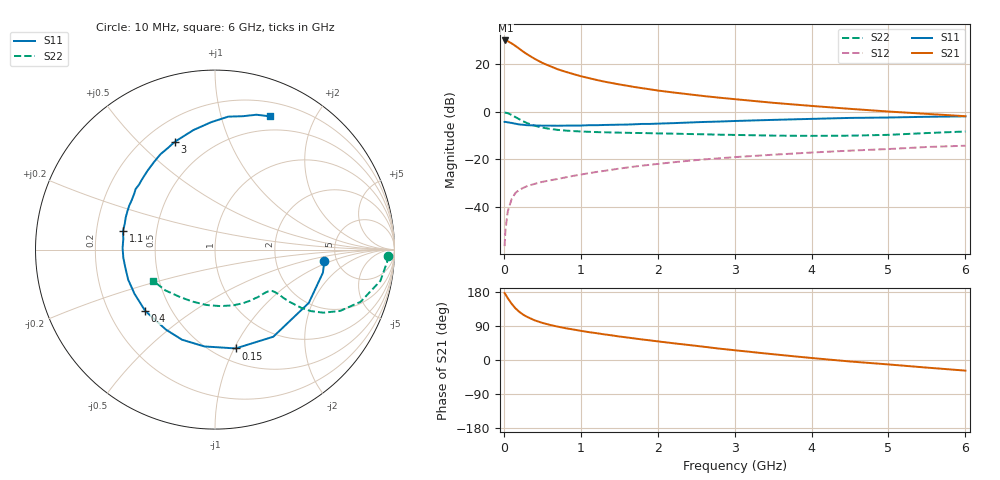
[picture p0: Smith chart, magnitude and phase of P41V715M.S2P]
! SIEMENS Small Signal Semiconductors
! BFP182
! Si NPN RF Bipolar Junction Transistor in SOT143
! VCE = 1.75 V  IC = 15 mA
! Common Emitter S-Parameters:  March  1996
# GHz  S  MA  R  50
!  f  S11  S21  S12  S22
! GHz  MAG  ANG  MAG  ANG  MAG  ANG  MAG  ANG
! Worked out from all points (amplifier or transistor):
!   36 points, 10 MHz to 6 GHz, reference 50 ohm
!   highest |S21| = 30.0 dB at 20 MHz (marker M1)
!   |S21| within 3 dB of that: start of sweep to 180.4 MHz
!   unconditionally stable (mu >= 1): 786.2 MHz to 5.449 GHz
!   at 250 MHz: K = 0.46, MSG = 28.7 dB, |S12| = -32.0 dB
!   at 1.4 GHz: K = 1.19, MAG = 15.6 dB, |S12| = -24.4 dB
!   at 6 GHz: K = 0.95, MSG = 6.2 dB, |S12| = -14.2 dB
!   S11 on the Smith chart (normalised r, x): 10 MHz: 3.98, -0.84; 150 MHz: 0.63, -1.01; 400 MHz: 0.36, -0.33; 1.1 GHz: 0.32, +0.09; 3 GHz: 0.32, +0.65; 6 GHz: 0.34, +1.44
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0.01  0.6128 -6.2  31.32 176.6  0.0015 78.2  0.9645 -2.0
0.02  0.6148 -12.1  31.61 173.6  0.0031 80.5  0.9607 -4.3
0.05  0.6011 -29.6  30.59 163.4  0.0079 81.9  0.9378 -10.7
0.1  0.5841 -56.2  27.52 148.8  0.0145 65.7  0.862 -19.7
0.15  0.5625 -78.2  24.32 136.6  0.0197 58.7  0.7766 -26.1
0.2  0.5428 -96.3  21.22 127.3  0.0229 54.4  0.699 -30.2
0.25  0.5346 -110.1  18.49 119.8  0.0251 50.8  0.6342 -32.7
0.3  0.5231 -121.4  16.32 114.1  0.0273 49.1  0.5809 -34.0
0.4  0.5175 -138.7  13.01 104.7  0.0306 47.7  0.5099 -35.0
0.5  0.5117 -151.2  10.69 98.0  0.0337 46.2  0.4659 -35.2
0.6  0.5119 -160.9  9.129 92.6  0.0363 46.8  0.4369 -35.1
0.7  0.5096 -168.4  7.849 88.1  0.0388 48.1  0.417 -35.2
0.8  0.5128 -175.0  6.963 84.0  0.0418 48.9  0.4037 -35.5
1  0.5142 173.3  5.606 77.0  0.0479 49.7  0.3862 -36.6
1.1  0.5231 168.6  5.134 73.7  0.0512 49.9  0.3805 -37.5
1.5  0.537 152.9  3.765 62.0  0.064 50.3  0.3654 -42.2
2.2  0.5778 130.7  2.554 44.3  0.0869 47.3  0.3479 -54.1
3  0.6413 110.4  1.846 25.8  0.1116 41.4  0.327 -71.8
3.5  0.6769 100.2  1.547 15.2  0.1254 37.2  0.3161 -84.7
4.5  0.7445 84.3  1.155 -3.9  0.1527 29.0  0.3153 -113.1
5.5  0.7862 72.9  0.905 -20.1  0.1822 20.9  0.3579 -140.6
6  0.8036 67.4  0.809 -28.0  0.1939 15.8  0.3859 -153.2
